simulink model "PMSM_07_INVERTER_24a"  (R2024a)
settings: Solver=VariableStepAuto  StartTime=0.0  StopTime=0.1  MaxStep=1e-6  RelTol=1e-5  AbsTol=1e-6  EnableMultiTasking=on
libraries: spsIGBTDiodeLib x6, spsSeriesRLCBranchLib x5, spsCurrentMeasurementLib x3, spsVoltageMeasurementLib x3, spsDCVoltageSourceLib x1, simulink x1, spspowerguiLib x1

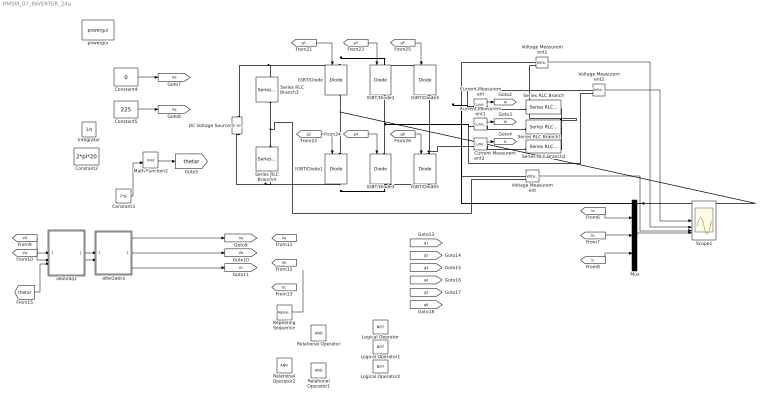
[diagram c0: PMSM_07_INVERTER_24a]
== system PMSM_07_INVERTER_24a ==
  Constant2 : Constant  Value=2*pi*20
  Constant3 : Constant  Value=2*pi
  Constant4 : Constant  Value=0
  Constant5 : Constant  Value=225
  Current Measurement : spsCurrentMeasurementLib/Current Measurement  PhasorSimulation=off  OutputType=Complex  PSBequivalent=0
  Current Measurement1 : spsCurrentMeasurementLib/Current Measurement  PhasorSimulation=off  OutputType=Complex  PSBequivalent=0
  Current Measurement2 : spsCurrentMeasurementLib/Current Measurement  PhasorSimulation=off  OutputType=Complex  PSBequivalent=0
  DC Voltage Source : spsDCVoltageSourceLib/DC Voltage Source  Amplitude=400  Measurements=None
  IGBT/Diode{,1..5} (6 alike) : spsIGBTDiodeLib/IGBT//Diode  Ron=1e-3  Rs=1e5  Cs=inf  Measurements=on
  Integrator : Integrator
  Logical Operator : Logic  Operator=NOT  AllPortsSameDT=off  OutDataTypeStr=boolean
  Logical Operator1 : Logic  Operator=NOT  AllPortsSameDT=off  OutDataTypeStr=boolean
  Logical Operator2 : Logic  Operator=NOT  AllPortsSameDT=off  OutDataTypeStr=boolean
  Math Function2 : Math  Operator=mod  SignedPower=on
  Mux : Mux  Inputs=3
  Relational Operator : RelationalOperator  OutDataTypeStr=boolean  RndMeth=Simplest
  Relational Operator1 : RelationalOperator  OutDataTypeStr=boolean  RndMeth=Simplest
  Relational Operator2 : RelationalOperator  OutDataTypeStr=boolean  RndMeth=Simplest
  Repeating Sequence : simulink/Sources/Repeating Sequence  rep_seq_t=[0 0.00005 0.0001]  rep_seq_y=[-200 200 -200]
  Scope1 : Scope  NumInputPorts=4
  Series RLC Branch : spsSeriesRLCBranchLib/Series RLC Branch  LConnTagsString=__new0  RConnTagsString=__new0  BranchType=RL  Resistance=10  Inductance=1e-3  SetiL0=off  InitialCurrent=0  Capacitance=1e-6  Setx0=off  InitialVoltage=0  Measurements=None
  Series RLC Branch1 : spsSeriesRLCBranchLib/Series RLC Branch  LConnTagsString=__new0  RConnTagsString=__new0  BranchType=RL  Resistance=10  Inductance=1e-3  SetiL0=off  InitialCurrent=0  Capacitance=1e-6  Setx0=off  InitialVoltage=0  Measurements=None
  Series RLC Branch2 : spsSeriesRLCBranchLib/Series RLC Branch  LConnTagsString=__new0  RConnTagsString=__new0  BranchType=RL  Resistance=10  Inductance=1e-3  SetiL0=off  InitialCurrent=0  Capacitance=1e-6  Setx0=off  InitialVoltage=0  Measurements=None
  Series RLC Branch3 : spsSeriesRLCBranchLib/Series RLC Branch  LConnTagsString=__new0  RConnTagsString=__new0  BranchType=RC  Resistance=1.e-3  Inductance=1e-3  SetiL0=off  InitialCurrent=0  Capacitance=470.e-6  Setx0=on  InitialVoltage=200  Measurements=None
  Series RLC Branch4 : spsSeriesRLCBranchLib/Series RLC Branch  LConnTagsString=__new0  RConnTagsString=__new0  BranchType=RC  Resistance=1.e-3  Inductance=1e-3  SetiL0=off  InitialCurrent=0  Capacitance=470.e-6  Setx0=on  InitialVoltage=200  Measurements=None
  Voltage Measurement : spsVoltageMeasurementLib/Voltage Measurement  PhasorSimulation=off  OutputType=Complex  PSBequivalent=0
  Voltage Measurement1 : spsVoltageMeasurementLib/Voltage Measurement  PhasorSimulation=off  OutputType=Complex  PSBequivalent=0
  Voltage Measurement2 : spsVoltageMeasurementLib/Voltage Measurement  PhasorSimulation=off  OutputType=Complex  PSBequivalent=0
  albe2abcs : Subsystem
  albe2dq1 : Subsystem
  powergui : spspowerguiLib/powergui  Priority=1  SimulationMode=Continuous  SampleTime=50e-6  frequency=60  Iterations=50  frequencyindice=0  Pbase=100e6  ErrMax=1e-4  UnitsV=kV  UnitsW=MW  buscounter=0  FunctionMessages=off  echomessages=off  EnableUseOfTLC=off  CurrentSourceSwitches=off  DisableSnubberDevices=on  DisableRonSwitches=on  DisableVfSwitches=on  DisplayEquations=off  AutomaticDiscreteSolvers=off  SolverType=Tustin  Interpol=off  ExternalGateDelay=off  methode=off  Ts=0  x0status=blocks  SPID=on  SwTol=0  HookPort=off  NonlinearTolerance=1e-4  nMaxIteration=100  ContinueOnMaxIteration=off  RestoreLinks=warning  ResistiveCurrentMeasurement=off  Frange=[0:2:500]  Ylog=off  Xlog=on  ShowGrid=off  save=off  variable=ZData  structure=0  ZoomFFT=off  StartTime=0.0  cycles=1  DisplayStyle=1  fundamental=60  FreqAxis=off  MaxFrequency=1000  frequencyindicesteady=1  RmsSteady=1  display=off
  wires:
  Mux/1 -> Scope1/4
  [Ia] -> Mux/1
  [Ib] -> Mux/2
  [Ic] -> Mux/3
  albe2dq1/1(alpha) -> albe2abcs/1(alpha)
  albe2dq1/2(beta) -> albe2abcs/2(beta)
  [Vc] -> ?
  [Vb] -> ?
  [Va] -> ?
  [Vq] -> albe2dq1/2(q)
  [Vd] -> albe2dq1/1(d)
  [thetar] -> albe2dq1/3(thetar)
  [g1] -> IGBT/Diode/1
  [g2] -> IGBT/Diode1/1
  [g3] -> IGBT/Diode2/1
  [g4] -> IGBT/Diode3/1
  [g5] -> IGBT/Diode4/1
  [g6] -> IGBT/Diode5/1
  Repeating Sequence/1 -> ?
  ? -> [g1]
  ? -> [g2]
  ? -> [g4]
  ? -> [g3]
  ? -> [g5]
  ? -> [g6]
  Constant2/1 -> ?
  ? -> Math Function2/1
  Constant3/1 -> Math Function2/2
  Math Function2/1 -> [thetar]
  Constant5/1 -> [Vq]
  Constant4/1 -> [Vd]
  Current Measurement/1 -> [Ia]
  Current Measurement1/1 -> [Ib]
  Current Measurement2/1 -> [Ic]
  Voltage Measurement/1 -> Scope1/3
  Voltage Measurement1/1 -> Scope1/2
  Voltage Measurement2/1 -> Scope1/1
  albe2abcs/1(as) -> [Va]
  albe2abcs/3(cs) -> [Vc]
  albe2abcs/2(bs) -> [Vb]
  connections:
  IGBT/Diode1/LConn1 -- Voltage Measurement2/LConn1 -- Current Measurement/LConn1 -- Voltage Measurement1/LConn1 -- Voltage Measurement/LConn1 -- IGBT/Diode/RConn1
  IGBT/Diode3/LConn1 -- Voltage Measurement2/LConn2 -- Current Measurement1/LConn1 -- IGBT/Diode2/RConn1
  IGBT/Diode5/LConn1 -- Current Measurement2/LConn1 -- IGBT/Diode4/RConn1
  DC Voltage Source/RConn1 -- IGBT/Diode4/LConn1 -- IGBT/Diode2/LConn1 -- IGBT/Diode/LConn1 -- Series RLC Branch3/LConn1
  IGBT/Diode1/RConn1 -- IGBT/Diode5/RConn1 -- IGBT/Diode3/RConn1 -- Series RLC Branch4/RConn1 -- DC Voltage Source/LConn1
  Series RLC Branch/RConn1 -- Voltage Measurement1/LConn2 -- Series RLC Branch2/RConn1 -- Series RLC Branch1/RConn1
  Current Measurement2/RConn1 -- Series RLC Branch2/LConn1
  Current Measurement1/RConn1 -- Series RLC Branch1/LConn1
  Current Measurement/RConn1 -- Series RLC Branch/LConn1
  Series RLC Branch4/LConn1 -- Voltage Measurement/LConn2 -- Series RLC Branch3/RConn1

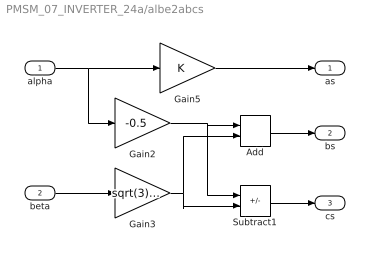
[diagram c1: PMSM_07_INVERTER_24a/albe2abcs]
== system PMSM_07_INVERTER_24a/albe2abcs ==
  alpha : Inport
  beta : Inport  Port=2
  Add : Sum
  Gain2 : Gain  Gain=-0.5
  Gain3 : Gain  Gain=sqrt(3)/2
  Gain5 : Gain
  Subtract1 : Sum  Inputs=+-
  as : Outport
  bs : Outport  Port=2
  cs : Outport  Port=3
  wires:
  alpha/1 -> Gain2/1, Gain5/1
  Gain3/1 -> Subtract1/2, Add/2
  Gain2/1 -> Subtract1/1, Add/1
  Add/1 -> bs/1
  Subtract1/1 -> cs/1
  beta/1 -> Gain3/1
  Gain5/1 -> as/1

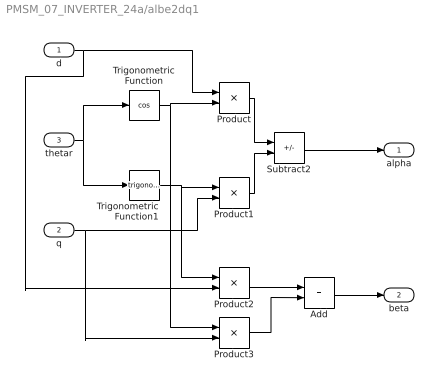
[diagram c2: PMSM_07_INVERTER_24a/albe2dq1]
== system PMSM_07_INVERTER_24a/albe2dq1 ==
  d : Inport
  q : Inport  Port=2
  thetar : Inport  Port=3
  Add : Sum
  Product{,1..3} (4 alike) : Product
  Subtract2 : Sum  Inputs=+-
  Trigonometric Function : Trigonometry  Operator=cos
  Trigonometric Function1 : Trigonometry
  alpha : Outport
  beta : Outport  Port=2
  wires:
  Product3/1 -> Add/2
  Product2/1 -> Add/1
  d/1 -> Product2/2, Product/1
  Add/1 -> beta/1
  Subtract2/1 -> alpha/1
  Product1/1 -> Subtract2/2
  Product/1 -> Subtract2/1
  q/1 -> Product1/2, Product3/2
  Trigonometric Function1/1 -> Product1/1, Product2/1
  Trigonometric Function/1 -> Product/2, Product3/1
  thetar/1 -> Trigonometric Function1/1, Trigonometric Function/1
